ORGANIZATION_BLOCK MAIN:OB1
TITLE=

BEGIN
NETWORK 1
LD I0.6
= Q0.0

NETWORK 2
LD I0.7
O M0.0
A I1.1
= M0.0

NETWORK 3
LD M0.0
O I1.0
A I0.0
A I0.2
A I0.4
O Q0.1
AN I0.5
AN M1.0
= Q0.1

NETWORK 4
LDN I0.5
A I0.1
AN I0.0
= Q0.2

NETWORK 5
LDN I0.5
A I0.3
AN I0.2
= Q0.3

NETWORK 6
LD I0.5
LD M1.0
A I1.0
OLD
= M1.0

NETWORK 7
LD Q0.0
= Q0.4

NETWORK 8
LD M0.0
= Q0.5

END_ORGANIZATION_BLOCK

